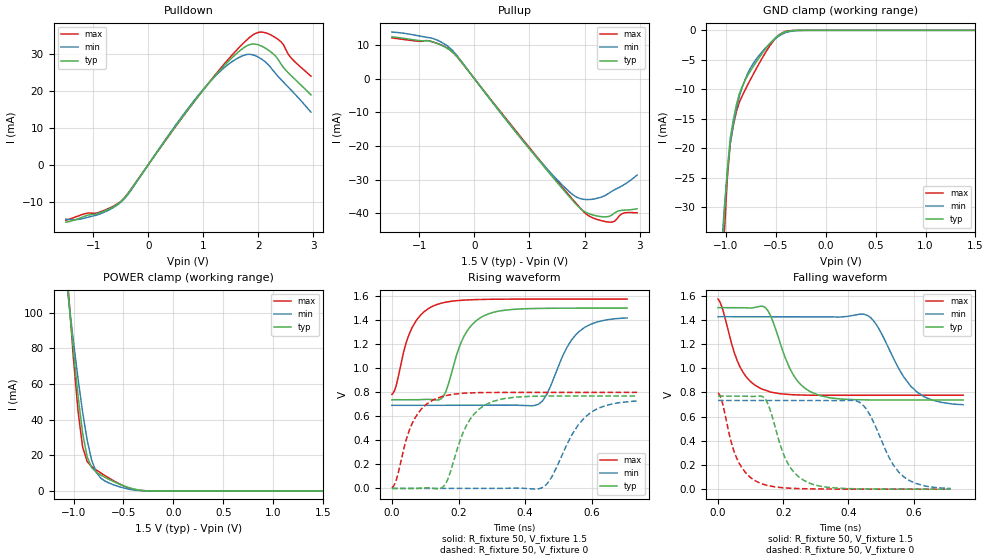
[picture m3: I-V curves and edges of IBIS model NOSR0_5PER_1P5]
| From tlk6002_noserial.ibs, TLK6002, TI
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[Model]   NOSR0_5PER_1P5
Model_type   3-state
Polarity   Non-Inverting
Enable   Active-Low
Cref =  15.0000pF
Rref =  100.0000M
Vref =  0V
Vmeas =  0.75
C_comp   2.108887p   1.924381p   2.428843p
[Temperature Range]   25   125   -40
[Voltage Range]   1.5   1.425   1.575
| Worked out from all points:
|   slope of the pulldown table from 0 to 0.225 V, typ, clamps not added: 47.1 ohm
|   slope of the pullup table from 0 to 0.225 V, typ, clamps not added: 47 ohm
|   GND clamp passes 1 mA (typ) near -0.48 V on its own axis
|   POWER clamp passes 1 mA (typ) near -0.39 V on its own axis
|   rising waveform, R_fixture 50, V_fixture 1.5: 20-80 % time 63.8ps typ, 76.1ps min, 58.3ps max; typ from 0.737 V to 1.5 V
|   rising waveform, R_fixture 50, V_fixture 0: 20-80 % time 67.9ps typ, 86.6ps min, 60.6ps max; typ from 0 V to 0.768 V
|   falling waveform, R_fixture 50, V_fixture 1.5: 20-80 % time 71.8ps typ, 91.4ps min, 62.7ps max; typ from 1.5 V to 0.738 V
|   falling waveform, R_fixture 50, V_fixture 0: 20-80 % time 64ps typ, 80.3ps min, 57.8ps max; typ from 0.769 V to 0.001 V
[POWER_clamp]
-1.5V     423.5mA    352.2mA    503mA
-1.061V   115.6mA    113mA      119.7mA
-1.045V   105.8mA    105.4mA    107.7mA
-1V       78.14mA    83.49mA    73.84mA
-954.5mV  53.09mA    62.89mA    44.72mA
-909.1mV  32.54mA    44.27mA    24.77mA
-863.6mV  19.13mA    28.63mA    16.48mA
-818.2mV  13.01mA    17.22mA    13.64mA
-772.7mV  10.47mA    10.51mA    11.79mA
-681.8mV  7.535mA    5.432mA    8.487mA
-318.2mV  297uA      112.4uA    206uA
1.5V      31.47nA    90.8nA     96.21nA
[Pulldown]
-1.5V     -15.59mA   -14.78mA   -15.08mA
-909.1mV  -13.19mA   -13.53mA   -12.99mA
-454.5mV  -9.369mA   -9.558mA   -9.315mA
909.1mV   18.53mA    18.79mA    18.54mA
1.318V    25.82mA    25.45mA    26.17mA
1.682V    31.06mA    29.27mA    32.21mA
1.909V    32.66mA    29.7mA     35.22mA
2.045V    32.18mA    28.69mA    35.89mA
2.182V    31mA       27.03mA    35.43mA
2.409V    27.27mA    23.05mA    33.28mA
2.591V    24.15mA    20.24mA    28.95mA
2.955V    18.91mA    14.22mA    23.95mA
[Pullup]
-1.5V     12.5mA     13.89mA    12.14mA
-772.7mV  11.03mA    12.06mA    11.02mA
-409.1mV  8.07mA     8.579mA    8.074mA
-227.3mV  4.842mA    4.968mA    4.737mA
1V        -20.87mA   -20.81mA   -20.52mA
1.5V      -30.8mA    -30.02mA   -30.43mA
1.818V    -36.84mA   -34.86mA   -36.55mA
2.091V    -40.22mA   -35.94mA   -40.93mA
2.409V    -41.07mA   -34.42mA   -42.6mA
2.545V    -39.94mA   -33.05mA   -42.43mA
2.727V    -39.1mA    -31.44mA   -39.92mA
2.955V    -38.69mA   -28.67mA   -39.87mA
[GND_clamp]
-1.5V     -337mA     -245.7mA   -453.6mA
-1.045V   -41.26mA   -37.73mA   -47.59mA
-1.015V   -31.48mA   -30.32mA   -34.73mA
-984.8mV  -23.81mA   -24.11mA   -25.24mA
-954.5mV  -18.25mA   -19.11mA   -19.1mA
-893.9mV  -12.68mA   -13.3mA    -13.81mA
-863.6mV  -10.74mA   -11.17mA   -12.17mA
-772.7mV  -7.41mA    -7.008mA   -8.983mA
-712.1mV  -5.806mA   -5.3mA     -7.048mA
-560.6mV  -2.304mA   -2.277mA   -2.676mA
-439.4mV  -510.4uA   -690.6uA   -461.1uA
1.5V      31.47nA    237.4nA    67.8nA
[Ramp]
dV/dt_f  0.3872744/57.07174p   0.3780456/75.94291p   0.4026931/49.32306p
dV/dt_r  0.3861834/53.58333p   0.3698341/70.54529p   0.4006777/47.52759p
R_load = 50
[Rising Waveform]
R_fixture = 50
V_fixture = 1.5
V_fixture_min = 1.425
V_fixture_max = 1.575
0s        737.4mV    691.4mV    782.7mV
60ps      737.2mV    691.4mV    1.334V
130ps     735.7mV    691.4mV    1.525V
162ps     805.6mV    691.4mV    1.549V
217ps     1.269V     691.4mV    1.567V
274ps     1.433V     691.3mV    1.572V
441ps     1.497V     702.4mV    1.575V
525ps     1.5V       1.171V     1.575V
561ps     1.5V       1.303V     1.575V
706ps     1.5V       1.418V     1.575V
[Rising Waveform]
R_fixture = 50
V_fixture = 0
V_fixture_min = 0
V_fixture_max = 0
0s        -2.254uV   1.073uV    5.259mV
12ps      -165.7nV   1.071uV    60.93mV
59ps      -182.8uV   1.061uV    529.8mV
125ps     600.9uV    1.047uV    738.3mV
166ps     65.22mV    -1.247uV   774.4mV
233ps     568.5mV    28.58uV    794.6mV
303ps     723.8mV    -541.8uV   798.4mV
450ps     767.8mV    4.561mV    798.6mV
578ps     768.5mV    588.5mV    798.9mV
736ps     768.4mV    726.4mV    799.2mV
[Falling Waveform]
R_fixture = 50
V_fixture = 1.5
V_fixture_min = 1.425
V_fixture_max = 1.575
0s        1.5V       1.425V     1.571V
66ps      1.5V       1.425V     1.018V
133ps     1.511V     1.425V     829.1mV
161ps     1.435V     1.425V     803.3mV
229ps     952.5mV    1.425V     780.9mV
283ps     805.9mV    1.425V     777mV
458ps     737.8mV    1.437V     776.6mV
569ps     737.2mV    929.8mV    776.6mV
610ps     737.3mV    803.6mV    776.6mV
752ps     737.5mV    698.6mV    776.6mV
[Falling Waveform]
R_fixture = 50
V_fixture = 0
V_fixture_min = 0
V_fixture_max = 0
0s        769.5mV    733.7mV    795.4mV
57ps      769.6mV    733.7mV    258.8mV
128ps     769.7mV    733.7mV    52.15mV
154ps     700.3mV    733.7mV    30.41mV
213ps     218.4mV    733.7mV    9.97mV
264ps     72.22mV    733.7mV    4.755mV
433ps     3.723mV    720mV      1.72mV
536ps     1.64mV     208mV      1.564mV
569ps     1.46mV     104.6mV    1.516mV
713ps     1.192mV    7.223mV    1.287mV
